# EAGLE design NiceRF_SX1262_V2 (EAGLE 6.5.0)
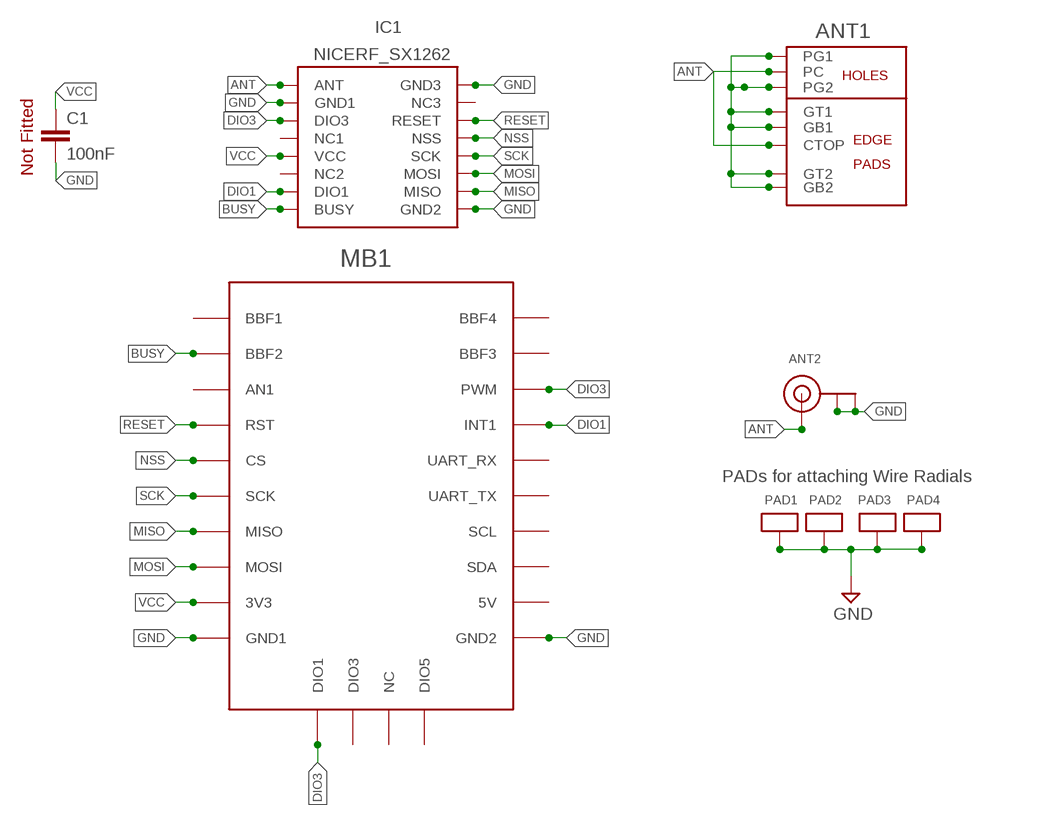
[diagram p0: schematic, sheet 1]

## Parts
ANT1  CUSTOMSMA  [CUSTOMSMA]
ANT2  ANTENNA_U.FL  [U.FL]
C1  100nF  C-EUC0805  [C0805]
IC1  NICERF_SX1262  [NICERF_SX1262]
MB1  BBFRIENDLY3  [PCB_SOCKET_BBFRIENDLY3]
PAD1  ANTPAD2  [ANTPAD2]
PAD2  ANTPAD2  [ANTPAD2]
PAD3  ANTPAD2  [ANTPAD2]
PAD4  ANTPAD2  [ANTPAD2]

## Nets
ANT: ANT1.CTOP ANT1.PC ANT2.3(SIGNAL) IC1.P$1(ANT)
BUSY: IC1.P$8(BUSY) MB1.BBF2
DIO1: IC1.P$7(DIO1) MB1.INT(INT1)
DIO3: IC1.P$3(DIO3) MB1.DIO1 MB1.PWM
GND [VDD]: ANT1.G1 ANT1.G2 ANT1.GB1 ANT1.GB2 ANT1.GT1 ANT1.GT2 ANT2.1(GND) ANT2.2(GND) C1.2 IC1.P$2(GND1) IC1.P$9(GND2) IC1.P$16(GND3) MB1.GND1 MB1.GND2 PAD1.P$1 PAD2.P$1 PAD3.P$1 PAD4.P$1
MISO: IC1.P$10(MISO) MB1.MISO
MOSI: IC1.P$11(MOSI) MB1.MOSI
NSS: IC1.P$13(NSS) MB1.CS
RESET: IC1.P$14(RESET) MB1.RST
SCK: IC1.P$12(SCK) MB1.SCK
VCC [VDD]: C1.1 IC1.P$5(VCC) MB1.3V3
Unconnected: IC1.P$4(NC1) IC1.P$6(NC2) IC1.P$15(NC3) MB1.5V MB1.AN1 MB1.BBF1 MB1.BBF3 MB1.BBF4 MB1.DIO3 MB1.DIO5 MB1.NC MB1.RX(UART_RX) MB1.SCL MB1.SDA MB1.TX(UART_TX)

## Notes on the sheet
- Not Fitted
- PADs for attaching Wire Radials

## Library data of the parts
ANT1 = con-coax:CUSTOMSMA
ANT2 = adafruit:ANTENNA_U.FL: U.FL Antenna Connector
C1 = resistor:C-EU: CAPACITOR, European symbol
IC1 = LMA2:NICERF_SX1262
MB1 = My_Mikrobus:BBFRIENDLY3
PAD1-PAD4 = LMA2:ANTPAD2

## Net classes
0 default: width 0.203 mm
1 POWER: width 0.635 mm
2 VDD: width 0.635 mm

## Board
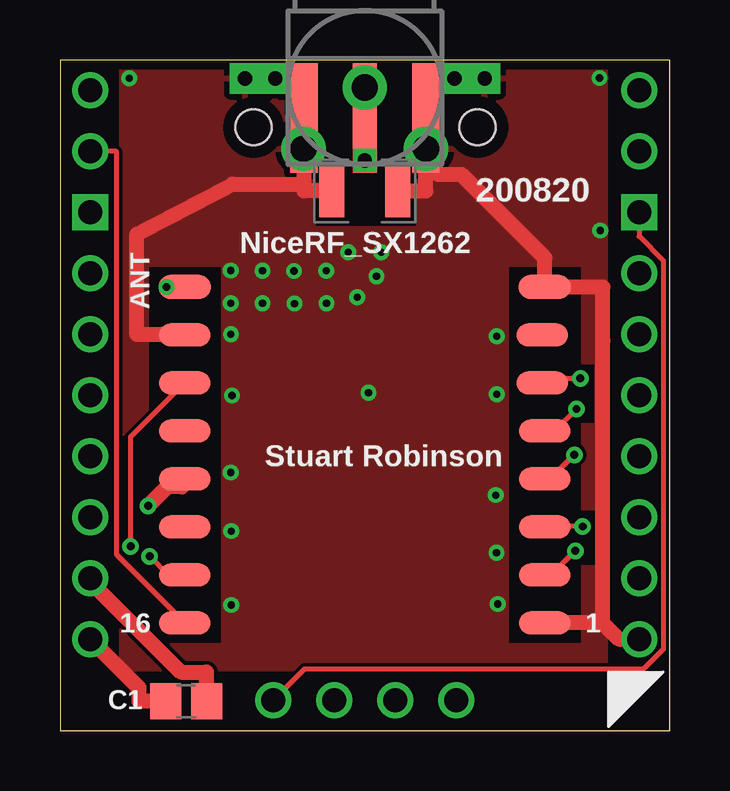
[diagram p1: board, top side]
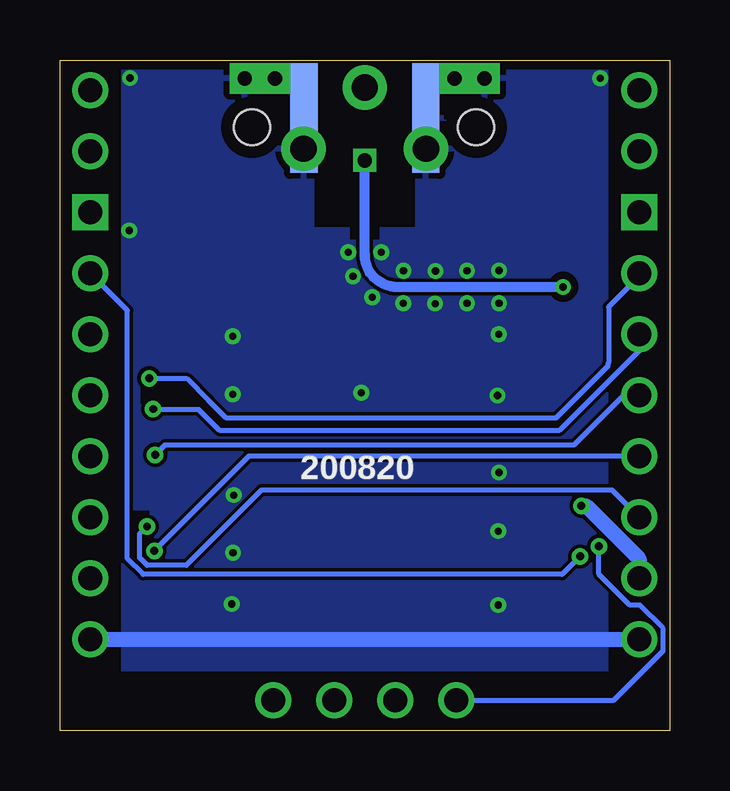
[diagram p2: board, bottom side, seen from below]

Size 25.4 x 27.94 mm. Coordinates in mm from the lower left corner, seen from the top.
Outline: 0,0 25.4,0 25.4,27.94 0,27.94 0,0
Copper layers (1*16): Top 0.0356mm / dielectric 1.5011mm / Bottom 0.0356mm
Design rules "LaenPCBOrder *": minimum track width 6mil, minimum drill 13mil, track to track 6mil, track to pad 6mil, pad to pad 6mil, via to via 6mil, smd to smd 6mil, copper to edge 15mil, drill to drill 6mil, minimum pad ring 7mil, minimum via ring 7mil, stop-mask expansion 4mil, vias tented up to drill 0mil, thermal gap 10mil
Holes 1.5 mm at 8.06,25.14 17.4,25.14
tRestrict: area 10.7,21 to 14.8,28.2; area 3.7,3.7 to 6.7,19.3; area 18.7,3.7 to 21.7,19.3; area 22.9,2.5 to 25.4,27.9; area 16.2,23.9 to 18.6,26.4; area 6.9,23.9 to 9.2,26.3; area 21.7,6.9 to 22.3,9.2; area 21.7,12.8 to 22.3,15.2; area 8.7,26.3 to 9.3,26.6; area 15.7,25.1 to 16.7,26.6
bRestrict: area 10.6,21 to 14.8,28.1; area 0,2.6 to 2.5,28; area 0,2.5 to 2.5,27.9; area 22.9,2.5 to 25.4,27.9; area 4,18.1 to 4.9,18.9; area 12.1,20.5 to 13.3,21; area 6.9,23.9 to 9.3,26.3; area 16.2,23.9 to 18.6,26.3; area 21.7,8.6 to 22.3,9.2; area 21.9,13.6 to 22,14.4; area 15.8,25.3 to 16.7,26.6; area 8.6,25.5 to 9.4,26.6

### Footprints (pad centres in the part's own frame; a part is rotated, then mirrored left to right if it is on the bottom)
CUSTOMSMA = smd 4.572 x 1.016: CTOP -1.27,0 | drill 1.1 pad 1.85: G1 -2.55,2.55; G2 -2.55,-2.55; PC 0,0 | smd 4.572 x 1.143 bottom: GB1 -1.27,2.54; GB2 -1.27,-2.54 | smd 4.572 x 1.143: GT1 -1.27,2.54; GT2 -1.27,-2.54
U.FL = smd 2.2 x 1.05: 1 0,1.375; 2 0,-1.375 | smd 0.8 x 1: 3 1.525,0
C0805 = smd 1.3 x 1.5: 1 -0.85,0; 2 0.85,0
NICERF_SX1262 = smd 2.2 x 1: P$1 -7.5,7.5; P$16 7.5,7.5 | smd 2.159 x 0.965: P$2 -7.5,5.5; P$3 -7.5,3.5; P$4 -7.5,1.5; P$5 -7.5,-0.5; P$6 -7.5,-2.5; P$7 -7.5,-4.5; P$8 -7.5,-6.5; P$9 7.5,-6.5; P$10 7.5,-4.5; P$11 7.5,-2.5; P$12 7.5,-0.5; P$13 7.5,1.5; P$14 7.4,3.5; P$15 7.4,5.5
PCB_SOCKET_BBFRIENDLY3 = drill 1: 3V3 -11.43,3.81; 5V 11.43,3.81; BBF1 -11.43,24.13; BBF2 -11.43,21.59; BBF3 11.43,21.59; BBF4 11.43,24.13; CS -11.43,13.97; DIO1 -3.81,-1.27; DIO3 -1.27,-1.27; DIO5 3.81,-1.27; GND1 -11.43,1.27; GND2 11.43,1.27; INT 11.43,16.51; MISO -11.43,8.89; MOSI -11.43,6.35; NC 1.27,-1.27; RST -11.43,16.51; RX 11.43,13.97; SCK -11.43,11.43; SCL 11.43,8.89; SDA 11.43,6.35; TX 11.43,11.43 | drill 1 square: AN1 -11.43,19.05; PWM 11.43,19.05
ANTPAD2 = drill 0.6 pad 1.27 square: P$1 0,0

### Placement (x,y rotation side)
ANT1  12.7,26.79 90 top
ANT2  12.7,22.49 90 top
C1  5.26,1.22 180 top
IC1  12.7,10.99 0 top
MB1  12.7,2.54 0 top
PAD1  8.97,27.17 0 top
PAD2  7.71,27.17 0 top
PAD3  16.44,27.17 0 top
PAD4  17.7,27.17 0 top

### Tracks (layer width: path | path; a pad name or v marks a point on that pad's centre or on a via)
ANT  (via drill 0.3, 0.6)
  Top 0.2: v12.7,23.76 ANT2.3
  Top 0.203: ANT1.PC 12.7,26.66 ANT1.CTOP
  Top 0.305: ANT1.PC ANT2.3
  Top 0.406: IC1.P$1 v4.44,18.48 | ANT1.CTOP ANT1.PC
  Bottom 0.406: v4.44,18.48 11.32,18.48 11.35,18.48 arc60 12.52,19.15 arc30 12.7,19.83 v12.7,23.76
BUSY
  Top 0.203: MB1.BBF2 2.35,24.13 2.35,7.34 IC1.P$8
DIO1  (via drill 0.33 pad 0.69)
  Top 0.203: v3.73,7.26 4.5,6.49 IC1.P$7
  Bottom 0.203: v3.73,7.26 4.48,6.51 21.93,6.51 22.59,7.17 22.59,17.51 MB1.INT
DIO3  (via drill 0.33 pad 0.69)
  Top 0.203: v2.94,7.68 2.94,12.23 IC1.P$3 | MB1.PWM 24.13,20.59 25.14,19.58 25.14,3.39 24.31,2.56 10.18,2.56 MB1.DIO1
  Bottom 0.203: MB1.DIO1 2.32,1.27 0.27,3.32 0.27,4.25 1.24,5.23 1.66,5.23 2.94,6.51 v2.94,7.68
GND  (via drill 0.3)
  Top 0.635: 22.6,4.49 23.28,3.81 MB1.GND2 | IC1.P$16 20.35,18.49 | 22.6,4.49 22.6,16.24 22.62,16.24 22.62,18.48 IC1.P$16 | 22.6,4.49 IC1.P$9 | IC1.P$16 20.2,19.7 16.73,23.16 15.74,23.16 15.24,23.66 15.24,24.18 ANT1.G2 | 5.08,16.5 IC1.P$2 5.08,16.5 | 10.16,22.76 7.19,22.76 3.2,20.68 3.2,16.5 3.64,16.5 5.08,16.5 | ANT1.GB2 ANT1.G2 | C1.2 3.29,1.22 3.29,1.79 MB1.GND1 | ANT1.G1 10.16,22.76 | ANT1.GB1 ANT1.G1 | 10.16,24.12 ANT1.G1 | ANT1.G1 | ANT2.2 15.25,22.49 ANT1.G2 | ANT2.1 10.16,22.49 10.16,22.76
  Bottom 0.635: MB1.GND2 MB1.GND1 | ANT1.GB2 ANT1.G2 15.24,24.12 | ANT1.GB1 ANT1.G1
  other vias: 2.89,27.18 7.14,8.31 18.19,7.41 18.24,5.27 7.14,5.23 7.17,13.96 7.12,16.51 18.2,14.01 18.2,16.43 7.11,10.75 18.16,9.81 7.11,19.17 7.11,17.8 8.44,19.16 8.44,17.8 9.75,19.15 9.77,17.79 11.09,19.16 11.1,17.8 12.01,19.93 13.39,19.93 12.39,18.05 13.19,18.93 22.48,27.19 22.51,20.84 12.85,14.08
  pour Bottom: 2.53,27.52 22.86,27.52 22.86,2.54 2.53,2.54
  pour Top: 2.54,27.5 22.86,27.5 22.86,2.54 2.54,2.54
MISO  (via drill 0.33 pad 0.69)
  Top 0.203: v21.47,7.49 20.47,6.49 IC1.P$10
  Bottom 0.203: MB1.MISO 17.53,11.43 v21.47,7.49
MOSI  (via drill 0.33 pad 0.69)
  Top 0.203: v21.78,8.5 20.21,8.5 IC1.P$11
  Bottom 0.203: MB1.MOSI 2.4,10.02 17.01,10.02 20.14,6.88 21.77,6.88 22.08,7.19 22.08,8.2 v21.78,8.5
NSS  (via drill 0.33 pad 0.69)
  Top 0.203: v21.52,13.4 20.61,12.49 IC1.P$13
  Bottom 0.203: MB1.CS 1.27,15.83 4.6,12.5 18.74,12.5 19.61,13.37 21.49,13.37 v21.52,13.4
RESET  (via drill 0.33 pad 0.69)
  Top 0.203: IC1.P$14 20.28,14.67 v21.68,14.67 | v21.68,14.67
  Bottom 0.203: MB1.RST 1.27,18.92 2.54,17.65 2.54,15.32 2.57,15.29 2.57,15.19 4.74,13.02 18.47,13.02 19.2,13.75 20.12,14.67 v21.68,14.67
SCK  (via drill 0.33 pad 0.69)
  Top 0.203: v21.43,11.49 20.43,10.49 IC1.P$12
  Bottom 0.203: 21.02,11.9 v21.43,11.49 21.03,11.89 3.99,11.89 1.91,13.97 MB1.SCK
VCC  (via drill 0.33 pad 0.69)
  Top 0.635: IC1.P$5 5.08,10.15 4.46,10.15 v3.67,9.36 | C1.1 6.11,2.44 5.03,2.44 1.27,6.2 MB1.3V3
  Bottom 0.635: v3.67,9.36 3.48,9.36 1.27,7.15 MB1.3V3

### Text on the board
tPlace: 200820 | NiceRF_SX1262 | ANT | Stuart Robinson | 16 | 1
bPlace: 200820
tNames: C1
